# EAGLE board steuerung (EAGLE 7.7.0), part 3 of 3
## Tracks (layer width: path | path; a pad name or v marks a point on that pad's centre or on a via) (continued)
N$170  (1 unrouted) (continued)
  Bottom 0.2: 13.8,17.7 14,17.9 14,17.5 13.3,18.7 | 13.3,18.5 13.3,17 | 13.3,17 13.3,16.2 | 18.6,14.6 17.9,14.6 17.8,14.7 | 18.6,14.6 18.7,14.6 | 18.7,14.6 IC4.8 18.7,14.4 19,14.4 | 13.2,18.6 13.2,18.9 13.3,18.7 | 13.2,18.6 13.3,18.5 | 13.3,18.5 13.3,18.7 | 13.3,18.7 14.1,17.57 14.1,19 | 19.4,14.4 19.2,14.4 19.2,14.6 18.7,14.6 | 18.2,14.8 18.3,14.7 | 13.8,17.7 13.6,18.8 | 13.6,18.8 13.5,18.7 13.5,18.6 | 13.6,18.3 13.5,18.2 | 13.5,18.2 13.6,18.1 | 13.6,18.3 13.6,17.8 13.5,17.7 13.4,17.7 13.5,17.6 | 13.6,18.3 13.7,18.4 | 13.5,17.2 13.4,17.3 13.5,17.4 13.5,17.5 13.7,17.5 14,17.2 | 13.4,16.9 13.3,17 | 13.5,16.6 13.4,16.7 | 13.4,16.4 13.4,16.3 | 13.3,18.7 13.8,17.7 | 13.2,18.6 13.2,17.97 | 18.6,14.6 18.6,14.2 18.5,14.1 | 17.7,14.1 17.5,14.1 17.25,13.85 | 32.5,15.7 32.5,18.1 32.7,17.6 32.2,19.1 | 32.5,15.7 32.8,15.7 | 32.9,15.7 33.2,15.7 | 33.2,15.7 37.9,15.7 38.8,14.8 38.8,12.6 | 38.8,12.6 39.2,12.6 | 39.2,12.6 41.4,12.6 | 41.4,12.6 41.4,13 | 41.4,13 41.4,13.7 | 39.1,14 41.4,14 41.4,13.7 | 39.1,14 38.9,14 38.9,12.7 39.5,12.7 40.8,13.1 | 40.8,13.1 39.5,13.9 39,13.9 39,13 39.1,12.9 39.3,12.9 39.3,13.8 39.1,13.8 39.1,12.8 | 39.1,12.8 39,12.8 | 39.1,12.8 39.4,12.8 | 39.4,12.8 40.8,13.1 | 40.8,13.1 41.2,13.1 C1.1 50.2,13.3 50.1,10.6 | 32.5,15.7 32.4,15.7 | 32.4,15.7 32.2,15.7 | 32.2,15.7 32.2,12.4 32.4,12.2 32.4,15.4 32.3,15.5 32.7,15.5 | 32.7,15.5 32.8,15.5 32.9,15.6 32.8,15.6 32.7,15.5 | 32.7,15.5 32.7,12.3 32.6,12.2 32.6,12.8 | 32.4,15.6 32.3,15.6 32.2,15.7 | 32.2,15.7 32.2,18.1 | 32.7,17.3 32.9,17.3 32.3,18.2 32.3,16.3 | 32.3,16.3 32.3,15.8 32.4,15.7 | 32.7,17.3 32.9,17.1 | 32.9,17.1 32.2,18.1 | 32.3,16.3 32.9,15.7 | 32.9,15.7 32.8,15.7 | 32.8,15.7 32.6,15.9
  Bottom 0.2: 32.6,15.9 37.5,15.9 | 37.7,15.9 37.9,15.9 | 37.9,15.9 38.9,14.9 38.9,14.2 39.1,14 | 50.3,16 55.7,16 | 55.7,16 55.8,16 | 55.8,16 55.9,15.9 55.9,15.2 | 55.9,15.2 55.9,14 | 55.9,14 55.9,13.1 | 55.9,13.1 55.9,13 | 55.9,13 54.5,13 | 54.5,13 54.5,13.1 | 54.5,13.1 54.5,13.6 52.8,15.3 | 52.8,15.3 52.7,15.3 | 41.2,13.8 41.1,13.9 41.1,13.8 41.3,13.6 41.4,13.7 | 50.5,15.6 50.6,15.6 | 50.6,15.6 50.8,15.8 50.4,15.8 50.3,15.4 | 50.3,15.4 50.8,15.4 50.9,15.5 50.7,15.5 50.6,15.6 | 50.6,15.6 51.62,15.6 IC1.16 52.55,15.76 53.1,15.2 | 53.5,14.8 54.5,13.8 54.5,14.4 | 54.5,14.6 54.5,15 | 54.5,15 54.5,15.8 54.4,15.9 | 54.4,15.9 52.8,15.9 | 54.4,15.9 55.4,15.9 | 55.4,15.9 55.6,15.9 | 55.6,15.9 55.7,15.9 55.8,15.8 | 55.8,15.8 55.6,15.8 | 55.6,15.8 52.9,15.8 52.8,15.7 53,15.5 55.8,15.5 55.8,15.7 | 55.8,15.7 55.6,15.7 | 55.6,15.7 53.2,15.7 53.1,15.6 53.1,15.4 54.4,14.1 54.4,14.3 53,15.7 55.4,15.7 55.7,15.4 | 55.7,15.4 53.6,15.4 53.5,15.3 53.6,15.2 54.5,15.2 | 55.8,15.2 55.9,15.2 | 55.9,15.2 55.7,15.4 | 55.7,15.4 55.7,15 55.8,14.9 55.5,14.9 | 55.5,14.9 54,14.9 53.8,15.1 55.7,15.1 55.8,15.2 | 55.8,15.2 54.5,15.2 | 54.5,15.2 54.1,14.8 54.2,14.8 54.4,14.6 | IC5.1 55.25,13.95 55.3,14 55.9,14 | 50.3,16 50.3,15.4 | 50.3,15.4 50.3,15.3 | 50.3,15.3 50.4,15.3 | 50.4,15.3 52.7,15.3 | 52.7,15.3 52.8,15.4 50.5,15.4 | 50.5,15.4 50.4,15.5 50.5,15.5 | 50.5,15.5 53.4,15.5 54.5,14.4 | 54.5,14.4 54.5,14.6 | 54.5,14.6 54.4,14.7 54.4,14.9 54.5,15 | 55.6,15.9 55.7,16 | 55.8,16 64.7,16 66,17.3 68,17.3 | 68,17.3 68.1,17.2 68.1,17.1 | 68.1,16.9 68.1,16.6 | 68.1,16.4 68.1,16.3 | 68.1,16.3 68.1,16 | 68.1,16 68.1,13.5 | 68.1,13.5 68.1,11.6 | 68.1,11.6 69.2,10.5 | 69.2,10.5 69.2,6.1 | 69.2,6.1 69.2,5.9
  Bottom 0.2: 69.2,5.9 69.2,1 | 69.2,0.8 69.2,0.5 | 69.2,0.5 69.2,0.4 68.8,0.4 | X2.1 45.08,5.92 45.72,5.92 50.1,10.5 | 50.1,10.5 50.2,10.6 50.1,10.6 | 45.4,5.7 45.4,5.8 45.8,6.2 | 45.8,6.2 46.1,6.5 | 46.1,6.5 50.1,10.6 | 50.1,10.6 50,10.7 45.6,6.3 | 45.8,6.2 45.8,5.7 | 45.8,5.7 45.7,5.6 | 54.6,13.7 54.6,13.2 54.5,13.1 | 54.5,13 54.5,12.6 55.9,12.6 55.9,13 | 55.9,13.1 54.9,13.1 54.6,12.8 55.8,12.8 | 68.3,0.4 53.5,0.4 | 53.5,0.4 53.3,0.4 | 53.3,0.4 22.6,0.4 20.4,0.3 20.1,3.4 20,3.5 20.1,2.9 20,4.3 18.7,5.5 | 18.7,5.5 17.8,6.4 17.8,8.1 16.9,9 16.9,13.5 17.25,13.85 | 17.3,14.1 17.2,14 17.2,13.9 17.25,13.85 | 16.7,8.9 17.6,8 17.6,6.3 18.6,5.3 | 18.6,5.3 19.7,4.3 19.6,3.4 19.7,3.1 | 19.7,3.1 19.5,3 19.9,0.5 20.5,0.2 | 20.5,0.2 20.7,0.2 | 20.7,0.2 69.2,0.2 | 69.2,0.2 69.4,0.4 | 69.4,0.4 69.4,10.6 68.3,11.7 68.3,13.3 68.1,13.5 | 68,17.3 68,17.2 | 68,17.2 68,11.7 68.1,11.6 | 69.2,10.5 69.3,10.5 69.3,10.6 68.2,11.7 | 55.4,15.9 55.6,15.7 | 55.8,15.7 64.8,15.7 66,16.9 68.1,16.9 | 68.1,16.9 68.1,17.1 | 68.1,17.1 68,17.2 | 68,17.2 66.1,17.2 66,17.1 | 66,17.1 67.6,17.1 | 67.6,17.1 67.9,17.1 | 67.6,17.1 67.6,16.9 68.1,16.4 | 68.1,16.4 68.1,16.6 | 68.1,16.6 67.9,16.8 | 66,17.1 65.1,16.2 | 65.1,16.2 64.7,15.8 | 64.6,15.8 55.8,15.8 | 55.6,15.8 55.6,15 55.5,14.9 | 55.5,14.9 55.5,15 56.4,15.9 | 65.1,16.2 67.9,16.2 68.1,16 | 68.1,16.3 65.6,16.3 66,16.7 67.7,16.7 67.7,16.6 67.9,16.4 66.2,16.4 | 65.6,16.4 66.2,16.4 | 66.2,16.4 66.3,16.5 67.7,16.5 67.8,16.6 65.8,16.6 65.7,16.5 | 19.9,1.2 20.7,1.2 20.7,0.2 | 20.5,0.2 19.1,0.2 19.1,0.9 | 19.1,0.9 20.5,0.9 20.5,0.5 19.3,0.5 19.3,0.4 | 19.3,0.4 19.2,0.4 | 19.3,0.4 20.3,0.4 | 20.3,0.4 20.3,0.7 19.5,0.7 | 19.5,0.7 19.2,0.7 19.2,0.6 19.5,0.6 19.5,0.7
  Bottom 0.2: 19.7,2.3 19.7,3.1 | 20.3,0.4 21,0.4 | 21.2,0.4 21.4,0.4 | 21.6,0.4 22.4,0.4 | 20.4,1.4 20.6,1.4 21.6,0.4 | 21.6,0.4 21.4,0.4 | 21.4,0.4 20.8,1 20.8,0.8 21.2,0.4 | 21.2,0.4 21,0.4 | 21,0.4 20.8,0.6 | 19.1,0.9 19.1,4.8 18.6,5.3 | 37.9,15.9 35.9,17.9 | 35.9,17.9 34.7,19.1 32.2,19.1 | 32.6,18.9 32.6,18.8 | 32.6,15.9 32.6,17.7 | 32.6,17.7 32.6,18.2 | 32.6,18.6 32.6,18.8 | 32.5,18.9 32.3,18.9 | 32.3,18.9 32.1,18.9 | 32,18.9 33.1,17.4 | 33,17.4 33.1,17.4 | 33.1,17.4 32.6,18.2 | 32.6,18.6 32.4,18.8 32.4,18.7 32.3,18.6 | 32.3,18.6 32.3,18.9 | 32.3,18.9 32.7,18.5 32.5,18.5 32.4,18.6 | 32.4,18.6 32.3,18.6 | 32.3,18.6 32.1,18.8 32.5,18.8 32.7,19 32.7,17.8 32.6,17.7 | 32.6,18.2 32.6,18.6 | 32.6,18.8 32.5,18.9 | 32.5,18.9 32.5,18 32.4,17.9 32.4,18.6 | 32.4,18.6 32.1,18.9 | 34.8,18.8 36.1,17.5 | 36.1,17.5 37.7,15.9 | 37.7,15.9 37.5,15.9 | 37.5,15.9 34.6,18.8 34.6,18.7 37.5,15.8 37.3,15.8 34.4,18.7 34.4,18.5 36.9,16 36.7,16 36.5,16.2 | 36,17.2 36,17.4 36.1,17.5 | 36.1,17.5 36.1,19.4 32.7,19.4 | 32.7,19.4 32.5,19.4 | 32.5,19.4 32.4,19.3 | 32.4,19.3 32.2,19.1 | 32.2,19.1 32,18.9 | 32,18.9 32.1,18.9 | 32.3,18.9 32.6,19.2 34.9,19.2 | 35.8,19.2 35.9,19.2 | 35.9,17.9 35.9,19.2 | 35.9,19.2 36,19.3 35.2,19.3 35,19.1 35.8,18.3 35.8,19.2 | 35.8,19.2 34.9,19.2 | 34.9,19.2 34.8,19.1 34.9,19.1 35.1,18.9 | 35.8,18.2 35.1,18.9 | 35.1,18.9 35.3,18.9 35.5,19.1 | 35.5,19.1 35.1,19.1 | 35.5,19.1 35.6,19.1 35.6,18.6 35.7,18.5 35.7,18.7 35.5,18.9 35.5,18.8 35.2,18.5 33.2,18.5 32.4,19.3 | 32.4,19.3 32.7,19.3 | 33.1,19.3 32.8,19.3 32.7,19.4 | 32.5,19.4 32.2,19.4 | 32.2,19.4 32.2,19.1 | 32.2,19.4 32,19.2 | 38.8,12.6 39.4,12.8 | 50.3,16 49.5,16 49.4,16.1 49.4,25.7 | 49.4,25.7 49.4,26.4 | 49.4,26.4 49.4,26.6
  Bottom 0.2: 49.4,26.6 49.3,26.6 | 49.3,26.6 48.2,26.6 | 48.2,26.6 48.1,26.5 | 48.1,26.5 48.1,26.4 | 48.1,26.4 48.1,22.11 | 48.1,22.11 48.1,21.5 | 48.1,21.5 48.1,15.9 | 48.1,15.9 48.1,15.7 | 48.1,15.7 48.1,15.6 | 48.1,15.6 48.1,15.4 | 48.1,15.4 48.1,15.2 | 48.1,15.2 53.1,15.2 | 53.1,15.2 53.5,14.8 | 53.5,14.8 53.4,14.8 52.9,15.3 52.8,15.3 | 49.8,15.3 49.4,15.3 49.3,15.4 49.3,15.5 | 49.3,15.7 49.3,15.9 49.8,15.9 | 49.8,15.9 50.1,15.9 50.2,15.8 50.2,15.6 50.1,15.5 | 50.1,15.5 49.3,15.5 | 49.3,15.5 49.3,15.7 | 49.3,15.7 49.4,15.8 | 49.4,15.8 49.8,15.8 | 49.8,15.8 50.1,15.5 | 50.1,15.5 50.1,15.8 49.8,15.8 | 49.4,15.8 49.6,15.6 50.4,15.6 50.5,15.5 | 50.5,15.5 50.5,15.4 | 50.5,15.4 50.4,15.3 | 50.3,15.3 49.8,15.3 | 49.8,15.3 49.5,15.6 50.1,15.6 50.3,15.4 | 48.3,26.2 48.1,26.4 | 48.1,26.5 48.1,26.6 | 48.6,26.3 48.4,26.3 48.1,26.6 | 48.1,26.6 48.2,26.6 | 49.3,26.5 49.3,26.6 | 49.4,26.6 54,26.6 54,26 49.9,26 49.3,25.4 49.3,25.7 49.8,26.2 49.9,26.2 | 49.9,26.2 53.8,26.2 53.9,26.1 53.9,26.3 49.8,26.3 | 49.8,26.3 49.5,26.3 49.4,26.4 | 49.4,26.4 49.7,26.4 | 53.9,26.4 49.7,26.4 | 49.7,26.4 49.3,26 49.3,25.8 49.8,26.3 | 49.8,26.3 49.9,26.2 | 49.9,26.2 49.4,25.7 | 65.6,0.3 68.5,0.3 69.2,1 | 69.2,1 69.2,0.8 | 69.2,0.8 69,0.6 | 69.3,6.3 69.3,6.2 69.2,6.1 | 69.2,6.1 68.9,5.8 68.9,1 68.3,0.4 | 68.3,0.4 68.8,0.4 | 68.8,0.4 69,0.6 | 69,0.6 69,5.7 69.2,5.9 | 68.5,0.5 68.6,0.5 | 68.6,0.5 69.2,0.5 | 53.3,0.4 53.6,0.7 68.8,0.7 68.9,0.6 68.7,0.6 68.6,0.5 | 68.5,0.5 53.6,0.5 53.5,0.4 | 39.2,12.6 39.7,13 39.4,12.8 | 44.7,5.4 44.5,5.4 44.2,5.7 44.2,6 | 44.2,6 44.2,6.2 45.3,6.2 | 45.3,6.2 45.8,6.2 | 45.8,5.7 45.8,5.5 44.7,5.5 44.4,5.8 | 44.4,5.8 44.2,6 | 44.2,6 44.4,6 | 44.4,6 45.7,6 45.7,5.9 45.6,5.8 44.4,5.8
  Bottom 0.2: 43.9,6.5 44.4,6 | 39.7,12.7 39.9,13.7 | 39.9,13.7 41.4,13 | 41.4,13 41.8,12.6 41.7,12.6 39.9,13.7 | 39.9,13.7 39.6,12.4 | 46.8,7.6 46.6,7.6 | 42.3,3 42.2,2.4 | 42.2,2.4 43.8,2.4 43.9,2.3 44.3,2.3 | 45.5,2.3 44.3,2.3 | 44.3,2.3 44.2,2.4 44,2.4 | 43.9,2.4 44,2.4 | 44,2.4 44.1,2.5 42.3,2.5 42.1,2.7 | 42.1,2.7 42.2,3 | 42.2,3 42.3,3 | 42.4,3 42.8,3 | 42.8,3 43.1,3 | 43.1,3 43.3,3 | 43.3,3 43.4,3 | 43.8,3 44.3,3 44.4,2.9 44.2,2.9 | 42.1,2.9 42.4,2.9 | 42.7,2.9 43,2.9 | 43.2,2.9 44.2,2.9 | 44.2,2.9 44.4,2.7 44.3,2.7 | 42.2,2.7 42.3,2.7 | 42.3,2.7 44.3,2.7 | 44.3,2.7 44.4,2.6 42.3,2.6 42.1,2.8 | 42.3,3.1 42.1,3.1 42.1,7.3 | 42.2,3 42.2,7.5 42.1,7.5 | 42.2,3 42.2,2.8 42.3,2.7 | 42.3,2.7 42.3,3 | 42.3,3 42.3,3.1 | 42.3,3.1 42.3,7.7 43.7,6.9 | 42.3,3.1 42.4,3 | 42.4,3 42.4,2.9 | 42.4,2.9 42.5,2.8 42.5,3 | 42.5,7.4 42.5,7.8 | 43,2.9 43.1,3 | 43.1,3 43.1,7.5 | 43.1,7.5 43,7.5 43,7.4 | 43,7.4 43,2.9 | 43,2.9 43.2,2.9 | 43.2,2.9 43.3,3 | 43.3,3 43.3,7.5 | 43.3,7.5 43.2,7.6 43.2,7.4 | 43.2,7.4 43.5,7.1 | 43.5,7.1 43.5,3.1 43.4,3 | 43.4,3 43.8,3 | 43.8,3 43.8,6.8 | 43.8,6.8 43.7,6.9 | 43.7,6.9 43.6,7 | 43.6,7 43.6,3.1 44.1,3.1 44.1,7.1 44.3,7.3 44.3,6.9 | 44.3,6.9 43.9,6.5 | 43.9,6.5 43.9,3.1 44.3,2.7 | 44.3,2.7 44.3,2.4 | 44.5,6.4 44.2,6.4 | 69.4,0.4 69.4,0.2 69.2,0.2 | JP4.2 49.63,10.97 50.1,10.5 | IC1.6 48.1,22.11 | 47.7,22 47.7,21.9 48.1,21.5 | IC1.1 48.7,15.76 48.7,15.7 48.1,15.7 | 47.9,15.4 48.1,15.4 | 48.1,15.2 47.9,15.4 | 48.1,15.6 43.4,15.6 43.2,15.8 48,15.8 48.1,15.9 | 49.2,16.6 49.2,16.5 49.8,15.9 | 32.6,17.5 32.7,17.5 32.7,17.9 | 32.7,18.1 32.7,19.4 | 32.9,18.1 32.7,17.3 | 32.9,17.1 33.1,17.1 32.7,19.4 | 32.2,19.4 32.9,17.9 32.7,18.1 | 32.7,18.1 32.7,17.9 | 32.7,17.9 32.8,17.8 33,17.8 33.1,17.7
  Bottom 0.2: 14.4,18.6 14.4,18.4 14.3,18.4 | 19.9,14.1 20,14.1 20,15 18.2,15 | 19.9,14.1 19.8,14.2 19.8,14.7 | 17.7,8.1 16.9,8.9 16.7,8.9 | 19.8,14.7 19.8,14.9 | 13.5,16.3 13.4,16.4 | 13.4,16.4 13.4,16.7 | 13.4,16.8 13.4,18.2 13.8,18.6 13.9,18.6 | 14.5,17.4 14.2,17.3 | 14.1,17.2 14.1,17.3 | 14.1,17.3 14.2,17.3 | 14.5,17.4 14.4,17.4 | 14.4,17.4 14.2,17.4 | 13.7,17.4 13.88,18.5 | 13.88,18.5 13.9,18.6 | 13.9,18.6 13.8,18.5 13.8,18.4 | 13.8,17.2 13.8,16.6 | 13.8,16.6 13.6,16.4 13.6,16.8 | 13.6,16.8 13.7,16.9 | 13.7,16.9 13.7,17 | 13.7,17.9 13.7,17 | 13.7,17 13.5,16.8 | 13.5,16.8 13.6,16.8 | 13.6,16.8 13.9,16.5 13.8,16.4 13.8,16.6 | 13.8,17.2 13.8,18.4 | 13.8,18.4 13.7,17.4 | 13.7,17.4 14.2,17.4 | 14.2,17.4 14.3,17.3 14.3,16.8 | 13.9,16.6 13.9,16.9 | 13.9,16.9 13.9,17.1 | 13.9,18.2 13.9,18.3 13.7,17.2 13.8,17.2 | 13.9,17.2 14,17.2 | 14.1,17.2 14.2,17.3 | 14.2,17.2 14.2,17.1 | 14.2,17.1 14.2,17 | 14.5,17.4 14.5,17.3 | 14.5,17.3 14.5,16 15.6,14.9 | 14,16.8 13.9,16.9 | 13.9,16.9 14,16.9 14.1,17 | 13.8,17.2 13.9,17.2 | 14,17.2 14.1,17.2 | 14.1,17.2 14.2,17.2 | 14.2,17.2 14.4,17.2 14.5,17.3 | 14,17.2 14,17.4 14.2,17.6 | 14.2,17.6 13.9,17.1 | 13.9,17.1 13.9,17.2 | 14.2,17.2 14,17 13.7,16.9 | 13.7,16.9 13.9,17.1 | 13.9,17.1 14,17.1 | 14,17.1 14.1,17.1 14.2,17 | 14.2,17 14.5,17.4 | 14.5,17.4 14.2,17.1 | 14.2,17.1 14.1,17 | 14.1,17 14,17.1 | 13.9,18.2 13.9,17.2 | 14.3,18.4 14.2,17.5 | 14.2,17.3 14.2,17.2 | 14.2,17.8 14.2,17.6 | 14.2,17.6 14.2,17.5 | 14.2,17.5 14.2,17.3 | 42.1,2.7 42.3,3 | 42.3,3 42.4,3 | 42.2,2.4 42.1,2.4 42.1,7.7 45.9,7.7 48.9,10.7 48.9,12.4 48.7,12.6 41.4,12.6 | 38.8,12.6 38.8,12.5 48.9,12.5 49,12.6 | 45.9,7.4 46,7.4 | 46,7.4 46.4,7.4 46.6,7.6 | 46.6,7.6 46.5,7.6 | 46.5,7.6 45.3,6.4
  Bottom 0.2: 45.3,6.4 45.2,6.3 45.2,6.5 | 45.2,6.5 45.2,7 45.7,7.5 42.6,7.5 42.5,7.4 | 42.5,7.4 42.5,3 | 42.5,3 42.4,2.9 | 42.4,2.9 42.7,2.9 | 42.7,2.9 42.8,3 | 42.8,4.1 42.8,7.3 42.9,7.4 42.7,7.4 42.7,3.1 42.8,3 | 42.8,3 42.8,4.1 | 42.8,4.1 45.2,6.5 | 45.2,6.5 45.5,6.5 45.7,6.7 | 45.7,6.7 46.3,7.3 46.3,7.2 45.3,6.2 | 45.3,6.2 45.3,6.4 | 45.3,6.7 45.3,7 45.7,7.4 | 45.7,7.4 45.9,7.4 | 45.7,7.4 45.3,7.4 | 45.3,7.4 44.7,7.4 | 44.4,7.4 43.9,7.4 | 43.9,7.4 43.6,7.1 43.9,7.1 | 45.6,7.1 43.9,7.1 | 43.9,7.1 43.8,7.2 | 43.8,7.2 44.1,7.2 | 46,7.2 44.1,7.2 | 44.1,7.2 43.7,6.8 45.4,6.8 | 45.4,6.8 45.8,6.8 45.9,6.7 | 45.9,6.7 44.5,6.7 44.3,6.9 | 44.3,6.9 44.6,6.9 | 44.7,6.9 45.6,6.9 | 45.6,6.9 45.7,7 | 45.7,7 45.7,6.7 | 45.2,6.5 43.8,6.5 43.7,6.4 45.3,6.4 | 45.3,6.4 45.3,6.7 | 45.3,6.7 45.4,6.8 | 49.1,12.7 49.1,12 | 49.1,12 49.1,11.9 | 49.1,11.8 49.1,10.9 | 49.1,10.9 49,10.8 49,11 | 49,11 49,12.1 | 49,12.1 49,12.2 48.8,12.4 | 48.8,12.4 48.4,12.8 48.4,12.7 49,12.1 | 49.1,10.9 49.1,10.8 | 49.1,10.8 48.8,10.5 | 48.8,10.5 48.8,10.7 | 48.8,10.9 48.8,11 | 48.8,11 48.8,12.2 | 48.8,12.4 48.8,12.7 48.9,12.8 | 48.3,12.7 48.8,12.2 | 48.8,12.2 49.1,11.9 | 49.2,12.7 49.2,11.7 | 49.2,11.7 49.2,10.9 49.1,10.8 | 49.4,12.7 49.4,10.9 | 49.7,11.4 49.7,11.3 | 49.7,11.3 49.6,11.2 | 49.7,12.6 49.7,11.4 | 49.7,11.4 49.8,11.3 | 49.8,11.2 49.8,12.4 50.2,12.8 50.2,10.8 | 13.5,18.2 13.9,18.2 | 13.5,16.8 13.4,16.8 | 13.4,16.8 13.4,16.7 | 44.6,6.9 44.7,6.9 | 44.7,6.9 44.7,7.1 | R5.1 20.78,21.28 21.5,22 21.5,22.1 14.9,22.1 | 14.9,22.1 14.5,22.1 | 14.5,22.1 14.3,22.1 | 14.3,22.1 14.1,22.3 | 14.1,22.3 21.5,22.3 21.5,20.6 | 21.5,20.5 21.5,20.3 21.3,20.4 | 21.1,20.3 20,20.4 | 20,20.4 20,22 15,22 | 15,22 14.4,22 14.3,22.1 | 14.1,22.3 14.1,19.3
  Bottom 0.2: 14.1,19.2 14.1,18.72 13.88,18.5 | 13.6,18.8 14.1,19.3 | 14.1,19.3 14.1,19.2 | 14.1,19.2 14,19.1 | 14,19.1 13.8,18.9 13.8,18.8 14,18.6 | 20,20.4 19.7,20.4 | 19.7,20.4 19.6,20.5 | 19.6,20.5 19.6,20.8 | 19.6,20.8 19.6,21.3 19,21.9 | 19,21.9 19.8,21.9 19.9,21.8 19.9,21.5 | 19.9,21.4 19.9,20.5 19.8,20.4 19.8,21.2 | 19.8,21.2 19.8,21.4 | 19.8,21.4 19.8,21.7 19.4,21.7 | 19.4,21.7 19.7,21.4 | 19.4,21.7 19.3,21.8 19.4,21.8 19.8,21.4 | 14.3,18.8 14,19.1 | 14,19.1 14,18 14.1,17.9 | 14.5,22.1 14.5,18.5 | 14.5,18.5 14.5,17.5 | 14.5,17.5 14.4,17.4 | 14.1,17.3 14.2,17.2 | 14.6,21.6 15,22 | 14.3,18.8 14.3,18.4 | 32.2,18.1 32.2,18.4 | 32.2,18.4 32.2,18.5 31.2,19.7 | 31.2,19.7 31.3,19.7 31.6,19.2 | 31.8,19 31.9,18.9 32.2,18.9 32.3,19 32.1,19.2 31.9,19.2 31.8,19.3 31.8,19.1 31.9,19 31.8,19 | 31.8,19 31.6,19.2 | 31.6,19.2 31.7,19.3 | 31.2,19.7 21.3,19.7 21.3,20.1 21.2,20.2 | 21.1,20.3 21.3,20.4 | 21.3,20.4 21.4,20.1 | 46,7.4 46,12.2 | 46,12.2 46,12.8 | 45.1,12.8 45.4,12.8 46,12.2 | 48.8,12.4 48.8,12.2 | 48.8,12.2 46.2,12.2 46.2,12 49.1,12 | 49.1,11.9 49.1,11.8 | 49.1,11.8 49.2,11.7 | 49.2,11.7 46.2,11.7 46.1,11.8 | 46.1,11.8 49.2,11.8 49.3,11.9 49.3,11.5 46.1,11.5 | 46.1,11.5 46.1,11.3 | 46.1,11.3 49.5,11.3 | 49.7,11.3 49.5,11.3 | 49.5,11.3 49.3,11.1 46.2,11.1 46.2,8.3 | 46.2,8.3 46.3,8.2 46.3,8.3 49,11 | 49,11 48.8,11 | 46.5,11 46.4,11 46.3,10.9 46.3,10.8 | 46.3,10.8 46.3,8.6 46.4,8.5 46.4,8.6 48.8,11 | 48.8,11 48.7,11 | 48.7,11 46.7,11 | 46.7,11 46.4,10.7 46.4,10.3 | 46.4,10.3 46.4,10.2 | 46.4,10 46.4,8.9 46.5,8.8 | 46.5,8.8 46.8,9.1 | 46.8,9.1 47,9.3 | 47.2,9.5 48.2,10.5 | 48.2,10.5 48.7,11 | 46.7,11 46.5,11 | 46.5,11 46.3,10.8 | 46.3,10.8 48.7,10.8 48.8,10.9 | 48.8,10.9 48.8,10.7
  Bottom 0.2: 48.8,10.7 48.7,10.6 46.6,10.6 46.5,10.7 46.5,10.4 46.4,10.3 | 46.4,10.3 46.9,10.3 | 47.2,10.3 48.6,10.3 48.8,10.5 | 48.8,10.5 48.2,10.5 | 48.2,10.5 46.6,10.5 46.6,9.9 | 46.6,9.6 46.6,9.1 | 46.6,9.1 46.6,9 46.5,8.9 46.5,9.9 46.9,10.3 | 46.9,10.3 46.9,10.2 | 46.9,9.3 46.9,10.2 | 46.9,10.2 46.7,10.4 46.7,9.2 46.8,9.1 | 46.8,9.1 46.8,9.3 47.4,9.9 | 47.4,9.9 47.9,10.4 47.6,10.4 | 47.6,10.4 47.4,10.4 | 47,10.4 46.9,10.3 | 46.9,10.3 47.2,10.3 | 47.2,10.3 47.2,9.5 | 47.2,9.5 47,9.3 | 47,9.7 47,10.4 | 47,10.4 47.4,10.4 | 47.4,10.4 47.4,10.2 | 47.4,9.9 47.4,10.2 | 47.4,10.2 47.6,10.4 | 45.3,7.4 46.2,8.3 | 43,7.4 43.6,7.4 46.4,10.2 | 46.4,10.2 46.4,10 | 46.4,10 43.7,7.3 | 43.7,7.3 44,7.3 46.6,9.9 | 46.6,9.9 46.6,9.6 | 46.6,9.6 44.4,7.4 | 44.4,7.4 44.7,7.4 | 44.7,7.4 47,9.7 | 47,9.7 47,9.3 | 46.5,8.8 45,7.3 45,7.5 46.6,9.1 | 46.6,9.1 46.3,9.1 44.5,7.3 44.5,7.7 46.8,10 46.5,10 43.9,7.4 | 21.4,20.7 21.5,20.6 | 21.5,20.6 21.5,20.5 | 21.5,20.5 21.2,20.2 | 30.8,19.8 32.2,18.4 | 14.7,14.8 16.5,14.8 16.55,14.75 | 16.55,14.75 16.8,14.5 | 14.2,17 14.2,16.9 14,16.7 | 16.9,15 15.3,15 | 15.3,15 15,15 14.8,15.2 14.8,15.1 14.9,15 14.8,14.9 15.2,14.9 | 15.6,14.9 18.1,14.9 18.2,15 | 18.2,15 16.9,15 | 16.9,15 16.7,14.8 16.7,14.6 17,14.3 17,14 17.1,14 | 17.3,14.2 17.5,14.4 17.5,14.5 17.7,14.7 | 17.7,14.7 16.8,14.7 17.2,14.3 17.3,14.4 | 17.3,14.4 17.5,14.6 17.2,14.6 | 17,14.6 17.2,14.6 | 17.2,14.6 17.3,14.5 17.3,14.4 | 17.3,14.4 17.3,14.2 | 17.3,14.2 17.1,14 | 17.1,14 17.3,14 17.4,14.1 | 16.7,8.9 16.7,14.5 16.5,14.7 16.55,14.7 16.55,14.75 | 17.2,14.5 17.3,14.4 | 15.6,14.9 15.2,14.9 | 15.2,14.9 14.8,15.3 14.9,15.4 | 14.9,15.4 14.8,15.5 | 14.9,15.4 15.1,15.2 15.2,15.2 15.2,15.1 15.3,15
  Bottom 0.2: 14.9,22.1 14.9,21.9 14.4,21.4 14.4,21.5 14.8,21.9 | 14.8,21.9 14.6,21.9 | 14.8,21.9 15,21.9 | 15,21.9 19,21.9 | 19.3,21.1 19.7,21.1 19.8,21.2 | 14.4,20.9 14.4,21.3 14.8,21.7 | 14.8,21.7 15,21.9 | 15,21.9 15,21.7 | 15,21.4 15,21.2 14.9,21.2 14.6,20.9 14.6,21.4 14.7,21.5 14.8,21.5 | 14.8,21.5 15,21.7 | 15,21.7 15,21.4 | 15,21.4 14.7,21.1 14.7,21.4 14.8,21.5 | 14.8,21.5 14.9,21.4 14.8,21.3 19.8,21.3 19.9,21.4 | 19.9,21.4 19.9,21.5 | 19.9,21.5 14.9,21.5 14.8,21.4 14.8,21.6 19.3,21.6 19.4,21.7 | 14.8,21.7 19.4,21.7 | 18.8,21.4 18.8,21.3 19.3,20.8 | 19.7,20.4 19.7,20.6 19.2,21.1 | 19.2,21.1 19.3,21.1 | 19.3,21.1 19.6,20.8 | 19.3,21.1 19.3,20.8 | 19.3,20.8 19.6,20.5 | 19.7,20.4 19.8,20.3 21.1,20.3 | 21.1,20.3 21.2,20.2
(copper drawn outside any net)
  shapes: Bottom area x35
